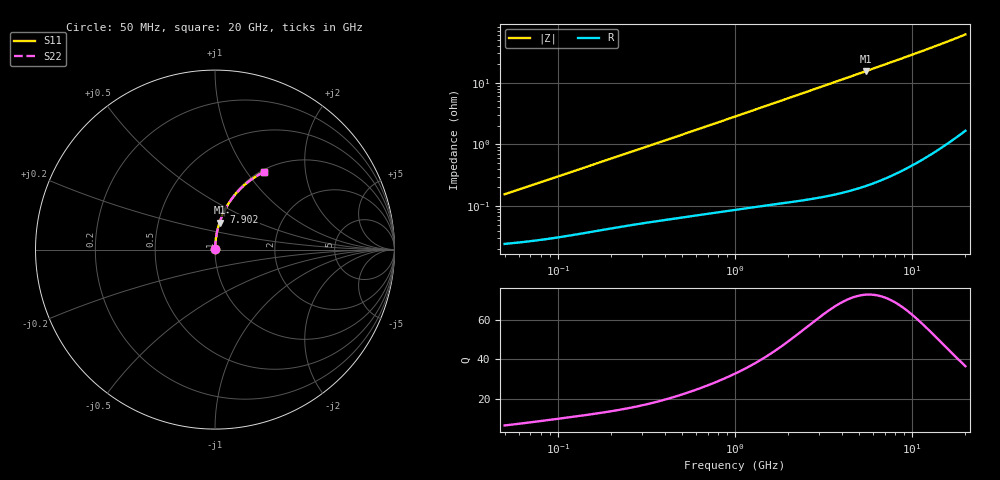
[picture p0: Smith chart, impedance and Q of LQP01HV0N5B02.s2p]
!Murata Part Number: LQP01HV0N5B02
!These Parameters are Measured in Series Mode Connection
!  o--[Z]--o
!Port1  Port2
!  o-------o
!Freq. Start=50[MHz] Stop=20[GHz], 401[Steps]
# Hz S RI R 50
!Freq.(Hz) S11(Real) S11(Imag) S21(Real) S21(Imag) S12(Real) S12(Imag) S22(Real) S22(Imag)
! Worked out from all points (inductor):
!   401 points, 50 MHz to 20 GHz, reference 50 ohm
!   read as one part in series: L = 483 pH near 51.52 MHz
!   highest Q = 73 at 5.516 GHz (marker M1), where L = 447 pH
!   S11 on the Smith chart (normalised r, x): 50 MHz: 1.00, +0.00; 7.902 GHz: 1.01, +0.45; 20 GHz: 1.03, +1.21
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5e7  0.000245 0.00153  0.9998 -0.00153  0.9998 -0.00153  0.000245 0.00153
5.152053e7  0.000247 0.00157  0.9998 -0.00157  0.9998 -0.00157  0.000247 0.00157
1.364002e8  0.000374 0.00404  0.9996 -0.00404  0.9996 -0.00404  0.000374 0.00404
3.721004e8  0.000687 0.0107  0.9993 -0.0107  0.9993 -0.0107  0.000687 0.0107
6.380365e8  0.00104 0.0181  0.999 -0.0181  0.999 -0.0181  0.00104 0.0181
1e9  0.00166 0.0281  0.9983 -0.0281  0.9983 -0.0281  0.00166 0.0281
1.714689e9  0.00337 0.0479  0.9966 -0.0479  0.9966 -0.0479  0.00337 0.0479
2.179053e9  0.00488 0.0607  0.9951 -0.0607  0.9951 -0.0607  0.00488 0.0607
2.728004e9  0.00708 0.0757  0.9929 -0.0757  0.9929 -0.0757  0.00708 0.0757
3.967106e9  0.0137 0.1094  0.9863 -0.1094  0.9863 -0.1094  0.0137 0.1094
5.515528e9  0.0254 0.1506  0.9746 -0.1506  0.9746 -0.1506  0.0254 0.1506
7.442007e9  0.0448 0.1999  0.9552 -0.1999  0.9552 -0.1999  0.0448 0.1999
7.901521e9  0.0502 0.2113  0.9498 -0.2113  0.9498 -0.2113  0.0502 0.2113
9.041845e9  0.0648 0.2388  0.9352 -0.2388  0.9352 -0.2388  0.0648 0.2388
1.034674e10  0.0837 0.2689  0.9163 -0.2689  0.9163 -0.2689  0.0837 0.2689
1.166392e10  0.1047 0.2976  0.8953 -0.2976  0.8953 -0.2976  0.1047 0.2976
1.295331e10  0.1272 0.3239  0.8728 -0.3239  0.8728 -0.3239  0.1272 0.3239
1.438523e10  0.1541 0.351  0.8459 -0.351  0.8459 -0.351  0.1541 0.351
1.597544e10  0.186 0.3782  0.814 -0.3782  0.814 -0.3782  0.186 0.3782
1.774144e10  0.2237 0.4047  0.7763 -0.4047  0.7763 -0.4047  0.2237 0.4047
1.940974e10  0.261 0.4261  0.739 -0.4261  0.739 -0.4261  0.261 0.4261
2e10  0.2745 0.4328  0.7255 -0.4328  0.7255 -0.4328  0.2745 0.4328
